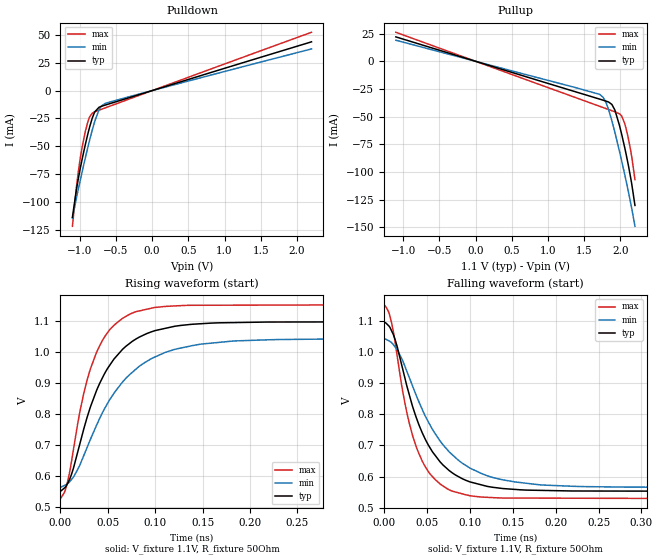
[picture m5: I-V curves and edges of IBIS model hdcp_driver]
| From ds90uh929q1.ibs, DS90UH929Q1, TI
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|   Model
[Model]   hdcp_driver
Model_type   Output
Polarity   Non-Inverting
Vmeas = 1
Vref = 1.1
Cref = 1pF
Rref = 50
|   typ   min   max
C_comp   0.756pF   0.476pF   0.975pF
[Voltage Range]   1.1   1.045   1.155
[Temperature Range]   27   105   -40
[Pullup Reference]   1.1   1.045   1.155
[Pulldown Reference]   0   0   0
[Power Clamp Reference]   1.1   1.045   1.155
[GND Clamp Reference]   0   0   0
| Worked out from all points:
|   slope of the pulldown table from 0 to 0.165 V, typ, clamps not added: 49.9 ohm
|   slope of the pullup table from 0 to 0.165 V, typ, clamps not added: 49.9 ohm
|   falling waveform, V_fixture 1.1V, R_fixture 50Ohm: 20-80 % time 43.4ps typ, 58ps min, 30.8ps max; typ from 1.1 V to 0.553 V
|   rising waveform, V_fixture 1.1V, R_fixture 50Ohm: 20-80 % time 42.9ps typ, 56.8ps min, 30.7ps max; typ from 0.551 V to 1.1 V
[Pulldown]
|   Voltage   I(typ)   I(min)   I(max)
-1.1V     -113.7mA   -114.5mA   -121.8mA
-1.037V   -86.09mA   -94.22mA   -82.7mA
-1.001V   -73mA      -83.23mA   -64.8mA
-961.4mV  -60.22mA   -71.65mA   -49.22mA
-892.1mV  -40.33mA   -52.33mA   -29.28mA
-859.1mV  -31.97mA   -43.65mA   -23.29mA
-826.1mV  -24.76mA   -35.44mA   -20.36mA
-789.8mV  -18.95mA   -27.25mA   -19.03mA
-733.7mV  -15.07mA   -17.45mA   -17.62mA
-694.1mV  -14.02mA   -13.55mA   -16.67mA
-644.6mV  -12.98mA   -11.42mA   -15.48mA
2.2V      43.7mA     37.34mA    52.27mA
[Pullup]
|   Voltage   I(typ)   I(min)   I(max)
-1.1V     22.1mA     19.09mA    26.27mA
1.715V    -34.19mA   -29.93mA   -40.68mA
1.761V    -35.11mA   -32.55mA   -41.77mA
1.801V    -35.93mA   -37.3mA    -42.71mA
1.883V    -39.16mA   -54.17mA   -44.66mA
1.926V    -44.71mA   -64.99mA   -45.69mA
1.986V    -57.74mA   -81.13mA   -47.4mA
2.018V    -66.48mA   -90.51mA   -49.65mA
2.058V    -77.85mA   -102.1mA   -56.14mA
2.111V    -94.59mA   -118.3mA   -70.3mA
2.157V    -111.5mA   -133.5mA   -86.86mA
2.2V      -130.2mA   -149.1mA   -106.9mA
[Ramp]
R_load = 50
|   typ   min   max
dV/dt_r   0.327324/4.25155e-11   0.28695/5.62998e-11   0.374488/3.06196e-11
dV/dt_f   0.327276/4.30029e-11   0.286867/5.75273e-11   0.374478/3.07078e-11
[Falling Waveform]
V_fixture = 1.1V
V_fixture_min = 1.045V
V_fixture_max = 1.155V
R_fixture = 50Ohm
C_fixture = 0F
|   Time   V(typ)   V(min)   V(max)
0s        1.098V     1.043V     1.153V
5.793ps   1.084V     1.037V     1.127V
9.167ps   1.067V     1.03V      1.092V
23.84ps   923.8mV    959.1mV    844.9mV
36.87ps   796.1mV    866.6mV    702.1mV
52.25ps   699.1mV    773.4mV    614mV
74.3ps    623.6mV    685mV      559.8mV
101ps     582.3mV    626.1mV    538.1mV
153.2ps   558.5mV    582.5mV    530.8mV
412.1ps   552.7mV    565mV      528.8mV
[Rising Waveform]
V_fixture = 1.1V
V_fixture_min = 1.045V
V_fixture_max = 1.155V
R_fixture = 50Ohm
C_fixture = 0F
|   Time   V(typ)   V(min)   V(max)
0s        551.4mV    564mV      527.9mV
6.836ps   573.2mV    574.4mV    573mV
11.55ps   605.1mV    589.2mV    645.4mV
23.84ps   743.1mV    660.8mV    856.1mV
38ps      875mV      763.4mV    998mV
52.25ps   958.1mV    847.2mV    1.072V
74.3ps    1.03V      930.2mV    1.123V
110.7ps   1.076V     998.5mV    1.146V
148ps     1.091V     1.025V     1.15V
412.1ps   1.097V     1.042V     1.152V
